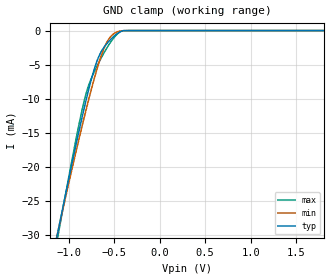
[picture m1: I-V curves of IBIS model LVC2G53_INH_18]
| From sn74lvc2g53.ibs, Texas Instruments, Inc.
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[Model]   LVC2G53_INH_18
Model_type  Input
Vinl=0.5775
Vinh=1.2675
| variable   typ   min   max
C_comp   3.45pF   2.97pF   4.06pF
[Temperature Range]   40   100   -40
| Ambient temperature   25   85   -40
[Voltage range]   1.8   1.65   1.95
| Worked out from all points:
|   GND clamp passes 1 mA (typ) near -0.52 V on its own axis
[GND Clamp]
| LVC2G53_INH_18
|   Voltage   I(typ)   I(min)   I(max)
-5.5V     -348.1mA   -320.8mA   -389.9mA
-1.145V   -31.41mA   -31.26mA   -32.35mA
-1.105V   -28.77mA   -28.83mA   -29.37mA
-905mV    -15.98mA   -17.05mA   -15.08mA
-840mV    -12.09mA   -13.41mA   -10.99mA
-800mV    -9.814mA   -11.25mA   -8.913mA
-720mV    -5.777mA   -7.161mA   -6.125mA
-665mV    -3.725mA   -4.658mA   -4.621mA
-585mV    -2.002mA   -1.855mA   -2.677mA
-505mV    -872.2uA   -477.4uA   -1.105mA
-390mV    -8.587uA   -16.56uA   -7.146uA
1.8V      127.5pA    516pA      1.129nA
